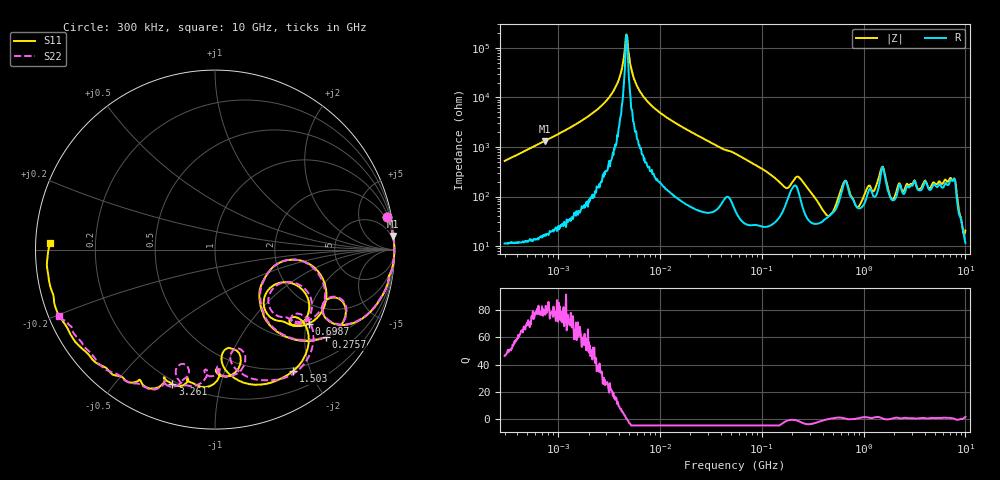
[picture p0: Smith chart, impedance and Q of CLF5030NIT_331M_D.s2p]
! S-Parameter Data Generated by TDK Corporation
! Copyright(C) 2019 TDK Corporation.
! All Rights Reserved.
! TDK P/N: CLF5030NIT-331M-D (Inductor)
! Property: L=330uH at 100kHz
! Size(LxWxT): 5.3x5x2.7mm
! Model Type: s2p (Touchstone File Format Version 1.0)
! Frequency: DC=Yes Start=0.3MHz Stop=10000MHz 802points Log-sweep
! Model Generated on May 10, 2019
! Port Assignments:
!  1 ---@@@--- 2
! Applicable Conditions:
!  Temperature = 25 degC
!  DC Bias Current = 0 A
!  Small Signal Operation
! Terms and conditions regarding TDK Simulation Models
! (1)This simulation model is being provided solely for informational purposes. Please refer to the specifications of the products in terms of detailed characteristics of such products.
! (2)In no event shall TDK Corporation of any of its subsidiaries be liable for any loss or damage arising, directly or indirectly,
!  From any information contained in this simulation model, including, but not limited to loss or damages arising from any inaccuracies, omissions or errors in connection with such information.
! (3)Any and all copyrights on this simulation model are owned by TDK Corporation.
!  Duplication or redistribution of this simulation model without prior written permission from TDK Corporation is prohibited.
! (4)This simulation model is subject to any modification or change without any prior notice.
! (5)Neither TDK Corporation nor any of its subsidiaries shall make any warranty, express or implied,
!  Including but not limited to the correctness, implied warranties of merchantability and fitness for a particular purpose with respect to this simulation models.
! (6)The use of this simulation model shall be deemed to have consented to the terms and conditions hereof.
# Hz S MA R 50
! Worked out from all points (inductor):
!   801 points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, 300 kHz to 10 GHz, reference 50 ohm
!   read as one part in series: L = 275 uH near 318.3 kHz
!   highest Q = 80.4 at 742.2 kHz (marker M1), where L = 282 uH
!   self-resonance near 4.673 MHz
!   S11 on the Smith chart (normalised r, x): 300 kHz: 1, +10; 275.7 MHz: 1.00, -2.54; 698.7 MHz: 1.40, -2.08; 1.503 GHz: 0.46, -1.75; 3.261 GHz: 0.18, -0.72; 10 GHz: 0.04, +0.02
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300000  0.9775 10.8  0.1873 -78.0  0.1873 -78.0  0.9773 10.8
742172  0.9957 4.3  0.07579 -84.9  0.07585 -84.9  0.9957 4.3
1713600  0.9989 1.6  0.02941 -87.3  0.02945 -87.4  0.999 1.6
3509086  0.9995 0.3  0.007454 -86.7  0.007449 -86.4  0.9996 0.3
4734969  0.9994 -0.2  0.0005415 7.9  0.0005053 11.6  0.9995 -0.2
6041662  0.9993 -0.6  0.006075 84.5  0.006165 84.6  0.9995 -0.6
9671944  0.999 -1.5  0.01909 86.3  0.0191 86.3  0.9991 -1.5
5.477226e7  0.9818 -9.8  0.1319 76.1  0.1319 76.1  0.9818 -9.8
2.756623e8  0.7866 -38.2  0.4628 38.8  0.4628 38.8  0.7873 -37.9
3.126428e8  0.7068 -46.0  0.5611 30.7  0.5611 30.7  0.7072 -45.7
4.269249e8  0.3843 -49.4  0.6991 -0.3  0.699 -0.3  0.3864 -48.8
5.414944e8  0.402 -8.6  0.6115 -30.6  0.6115 -30.6  0.3998 -8.5
6.987102e8  0.6663 -38.2  0.3532 -10.8  0.3531 -10.8  0.6604 -35.8
8.528959e8  0.421 -49.4  0.5814 -24.4  0.5814 -24.4  0.4339 -46.1
9.903836e8  0.4538 -23.9  0.5558 -52.0  0.5556 -52.0  0.4683 -22.9
1.307877e9  0.6197 -39.2  0.41 -72.7  0.4098 -72.7  0.6192 -36.7
1.50342e9  0.8045 -57.1  0.1693 -75.8  0.1692 -75.8  0.8144 -54.3
1.767019e9  0.7092 -82.6  0.3211 -39.9  0.3208 -39.9  0.7028 -78.2
3.261479e9  0.7865 -107.5  0.1574 -88.8  0.1569 -88.7  0.7472 -106.3
5.607117e9  0.8998 -130.3  0.08849 -141.1  0.08844 -140.2  0.8853 -125.2
7.652089e9  0.9418 -156.3  0.02393 -144.8  0.02522 -146.5  0.9138 -148.6
1e10  0.9207 177.9  0.04355 -101.2  0.04414 -100.9  0.9418 -157.0
